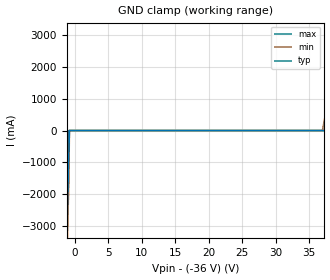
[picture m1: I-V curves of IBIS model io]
| TEXAS INSTRUMENTS INCORPORATED
| 1 Channel Uni-directional ESD-SURGE Protection Device
| Marketing Part #   Voltage Range   Package-type   #pins/pkg drawing
| TSD36-Q1   -36V-36V   SOD-323   2/DYF
[IBIS Ver]   4.1
[Comment char]  |_char
[File Name]   tsd36-q1.ibs
[File Rev]   1.0
"[Date]   Dec 20, 2023 "
[Source]   Data created from TI-SPICE simulations at TI-SLL/HVL.
   The following is an IBIS list for the TSD36.
   Please contact sllibis@ti.com with questions and
   comments concerning SLL IBIS models.
[Notes]
   - New measurements under nominal conditions only.
[Disclaimer]
"| TI and its licensors and suppliers make no warranties, either expressed"
"| or implied, with respect to this  model, including the warranties of "
"| provided solely on an ""as is"" basis. The entire risk as to its quality "
| and performance is with the customer.
[Copyright]
| (C) Copyright 2023 Texas Instruments Incorporated. All rights reserved.
| Component TSD36-Q1_DYF 2-PIN SOD-323
[Component]   TSD36-Q1_DYF
"[Manufacturer]   Texas Instruments, Inc."
[Package]   |2 SOD-323 - DYF package
   typ   min   max
R_pkg   23.0E-03   18.4E-03   27.6E-03
L_pkg   3.8E-10   3.04E-10   4.56E-10
C_pkg   5.7E-13   4.5E-13   6.8E-13
[Pin]   signal_name   model_name   R_pin   L_pin   C_pin
1   IO   io   2.07E-03   2.09E-10   6.95E-14
2   IO   io   2.07E-03   2.09E-10   6.95E-14
3   GND   gnd   2.07E-03   2.09E-10   6.95E-14
| Models and submodels in the file (1): io (Input)
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|   io Model
[Model]   io
Model_type  Input
| variable   typ   min   max
C_comp   16.5pF   13.2pF   19.8pF
[Voltage Range]   36   34   38
[Temperature Range]   27   -55   150
[Power Clamp Reference]   0   0   0
[GND Clamp Reference]   -36   -34   -38
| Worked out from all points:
|   GND clamp passes 1 mA (typ) near -0.80 V on its own axis
[GND Clamp]
|	Voltage  I(typ)   I(min)   I(max)
-3V       -18.3A     -19.2A     -17.5A
-1.3V     -4.17A     -5A        -3.33A
-1.1V     -2.5A      -3.33A     -1.67A
-900mV    -833mA     -1.67A     13.9fA
-800mV    -5nA       -5nA       -5nA
37V       4.63nA     4.63nA     4.63nA
39V       4.88nA     6.67A      4.88nA
40V       5nA        12.2A      5nA
41V       5.56A      17.8A      5.13nA
44V       22.2A      34.4A      5.5nA
45V       27.8A      40A        4.44A
50V       55.6A      67.8A      32.2A
[Power Clamp]
|   Voltage   I(typ)   I(min)   I(max)
-36V      0A         0A         0A
0V        0A         0A         0A
36V       0A         0A         0A
